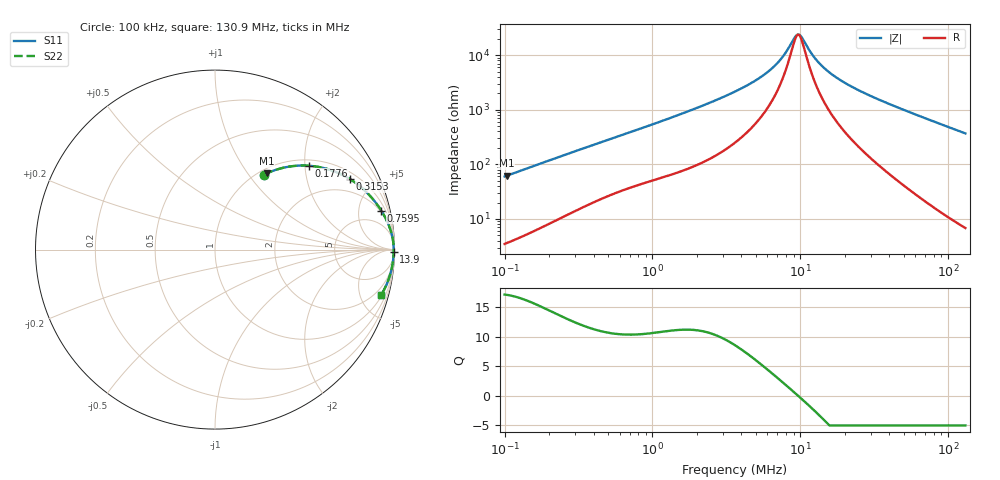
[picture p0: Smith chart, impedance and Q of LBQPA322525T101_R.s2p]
! LBQPA322525T101_R  S-PARAMETER MODEL  ( General Type )
! Model Generated by TAIYO YUDEN Corporation (http://www.ty-top.com)
! Version 1.0
! TAIYO YUDEN Control No. 191025NI43SB-FBB
! Copyright(c) 2019 TAIYO YUDEN CO.,LTD. All Rights Reserved.
! Product Description (link to TY-COMPAS)
! https://ds.yuden.co.jp/TYCOMPAS/or/detail?pn=LBQPA322525T101KR&u=M
! Products Name : Inductors
! Characteristics :
!  Inductance : 100 uH , SRF(min) : 6.0 MHz , DC Resistance(max) : 1.82 Ohm
!  Rated Current : Saturation :270 mA , Temp Rise : 220 mA (20 degC)
!  Case Size : 3.2 x 2.5 / 0.126 x 0.098 [mm/inch] , Thickness : 2.5 / 0.098 [mm/inch]
!  (Conditions: Temperature = 25 degC , DC Bias Current/Voltage = 0A / 0V)
! External Node Assignments :
!  1  o---GGG---o  2
! GND o---------o GND
! Frequency Range : 0.1MHz  -  130.914307MHz  [ 402 STEP ]
# MHz S RI R 50
! Freq[MHz].  S11 Real  S11 Imag  S21 Real  S21 Imag  S12 Real  S12 Imag  S22 Real  S22 Imag
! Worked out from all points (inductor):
!   401 points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, 100 kHz to 130.9 MHz, reference 50 ohm
!   read as one part in series: L = 94.6 uH near 103.7 kHz
!   highest Q = 17.1 at 103.7 kHz (marker M1), where L = 95 uH
!   self-resonance near 9.534 MHz
!   S11 on the Smith chart (normalised r, x): 100 kHz: 1.07, +1.19; 177.6 kHz: 1.14, +2.09; 315.3 kHz: 1.30, +3.63; 759.5 kHz: 1.80, +8.25; 13.9 MHz: open; 130.9 MHz: 1.14, -7.36
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0.1  0.2753 0.4184  0.7247 -0.4184  0.7247 -0.4184  0.2753 0.4184
0.103654  0.2887 0.4248  0.7113 -0.4248  0.7113 -0.4248  0.2887 0.4248
0.177566  0.5224 0.4673  0.4776 -0.4673  0.4776 -0.4673  0.5224 0.4673
0.315296  0.7507 0.3935  0.2493 -0.3935  0.2493 -0.3935  0.7507 0.3935
0.332733  0.7674 0.3827  0.2326 -0.3827  0.2326 -0.3827  0.7674 0.3827
0.484995  0.8599 0.3037  0.1401 -0.3037  0.1401 -0.3037  0.8599 0.3037
0.759537  0.9263 0.2174  0.0737 -0.2174  0.0737 -0.2174  0.9263 0.2174
1.10711  0.9585 0.1584  0.0415 -0.1584  0.0415 -0.1584  0.9585 0.1584
2.189296  0.9856 0.0819  0.0144 -0.0819  0.0144 -0.0819  0.9856 0.0819
3.683715  0.9927 0.0447  0.00735 -0.0447  0.00735 -0.0447  0.9927 0.0447
5.088039  0.9945 0.0275  0.00546 -0.0275  0.00546 -0.0275  0.9945 0.0275
6.424695  0.9953 0.0169  0.00472 -0.0169  0.00472 -0.0169  0.9953 0.0169
7.550657  0.9956 0.0101  0.00441 -0.0101  0.00441 -0.0101  0.9956 0.0101
9.03461  0.9958 0.00279  0.00422 -0.00279  0.00422 -0.00279  0.9958 0.00279
9.534256  0.9958 0.00063  0.00419 -0.00063  0.00419 -0.00063  0.9958 0.00063
10.2437  0.9958 -0.00224  0.00417 0.00224  0.00417 0.00224  0.9958 -0.00224
12.03896  0.9958 -0.00878  0.00419 0.00878  0.00419 0.00878  0.9958 -0.00878
13.89724  0.9957 -0.0148  0.0043 0.0148  0.0043 0.0148  0.9957 -0.0148
16.62851  0.9954 -0.0227  0.00458 0.0227  0.00458 0.0227  0.9954 -0.0227
20.62353  0.9948 -0.0332  0.00515 0.0332  0.00515 0.0332  0.9948 -0.0332
40.05754  0.9898 -0.0775  0.0102 0.0775  0.0102 0.0775  0.9898 -0.0775
130.9143  0.9273 -0.2506  0.0727 0.2506  0.0727 0.2506  0.9273 -0.2506
